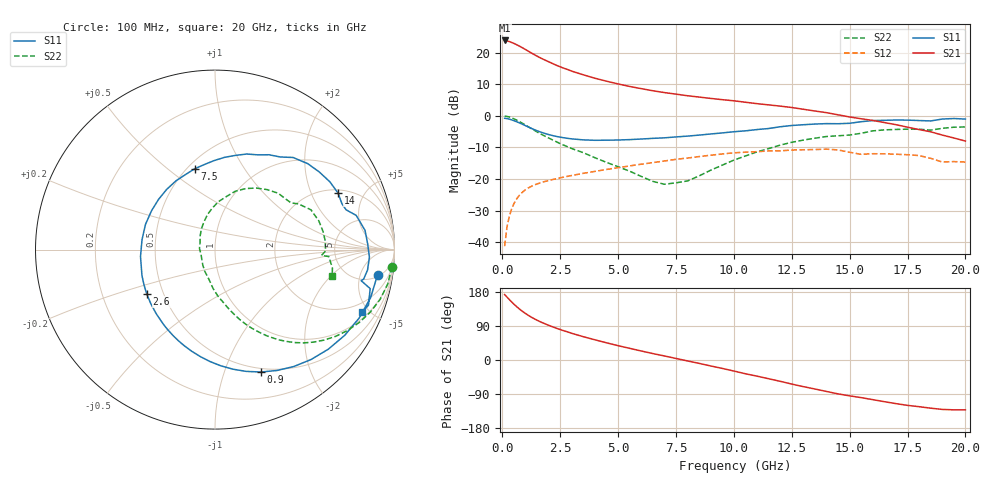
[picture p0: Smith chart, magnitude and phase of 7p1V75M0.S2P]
! Infineon Technologies  Discrete & RF Semiconductors
! bfp620
! VCE =  1.7 V,  IC =  5.0 mA
! Common Emitter S-Parameters:  Sep 2002
# GHz  S  MA  R  50
!  f  S11  S21  S12  S22
! GHz  MAG  ANG  MAG  ANG  MAG  ANG  MAG  ANG
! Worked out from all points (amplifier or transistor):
!   59 points, 100 MHz to 20 GHz, reference 50 ohm
!   highest |S21| = 23.9 dB at 100 MHz (marker M1)
!   |S21| within 3 dB of that: start of sweep to 1.03 GHz
!   unconditionally stable (mu >= 1): 4.847 GHz to 11.64 GHz; 14.74 GHz to 15.32 GHz; 17.15 GHz to end of sweep
!   at 1 GHz: K = 0.31, MSG = 22.2 dB, |S12| = -23.4 dB
!   at 5.5 GHz: K = 1.04, MAG = 11.4 dB, |S12| = -15.9 dB
!   at 20 GHz: K = 1.36, MAG = -0.3 dB, |S12| = -14.6 dB
!   S11 on the Smith chart (normalised r, x): 100 MHz: 6, -10; 900 MHz: 0.46, -1.34; 2.6 GHz: 0.40, -0.25; 7.5 GHz: 0.54, +0.62; 14 GHz: 2.17, +3.18; 20 GHz: 1.34, -4.53
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0.1  0.9165 -8.8  15.72 172.7  0.0086 80.6  0.9902 -5.6
0.2  0.9075 -17.1  15.49 166.2  0.0171 80.6  0.9816 -11.2
0.3  0.8892 -25.4  15.1 159.8  0.0253 76.8  0.9612 -16.7
0.4  0.8661 -33.5  14.63 153.5  0.0332 72.6  0.9332 -21.9
0.5  0.8406 -41.3  14.12 147.5  0.0404 68.6  0.9005 -26.8
0.7  0.7856 -56.0  13.01 136.6  0.053 61.3  0.8281 -35.7
0.9  0.7286 -69.4  11.86 127.1  0.0632 55.2  0.7531 -43.2
1.2  0.6479 -87.2  10.23 115.0  0.0747 47.9  0.6471 -52.2
1.4  0.6021 -97.7  9.29 108.2  0.0807 44.2  0.5854 -57.0
1.6  0.564 -107.3  8.492 102.1  0.0858 41.3  0.5321 -61.1
2  0.5065 -124.4  7.224 91.6  0.0945 36.9  0.4467 -67.8
2.6  0.4536 -147.0  5.805 78.3  0.1061 32.0  0.3506 -75.8
3.5  0.4168 -174.7  4.483 61.5  0.1229 26.2  0.2611 -86.2
5  0.4146 148.5  3.213 37.8  0.1512 17.2  0.1565 -105.2
7  0.4491 111.5  2.344 10.7  0.1928 3.7  0.0825 -160.7
7.5  0.4642 104.2  2.216 4.1  0.2051 -0.4  0.0869 175.5
10.5  0.5796 65.6  1.647 -36.3  0.266 -29.3  0.2317 93.8
12  0.6728 49.7  1.43 -56.2  0.2796 -44.0  0.3444 70.8
13.5  0.7429 30.6  1.196 -76.5  0.2928 -60.0  0.4428 49.0
14  0.7546 24.7  1.126 -83.0  0.2971 -66.3  0.4715 41.8
17  0.8614 -2.8  0.726 -115.1  0.2466 -90.7  0.6102 9.6
20  0.8908 -23.0  0.399 -131.6  0.1854 -104.8  0.6691 -12.5
